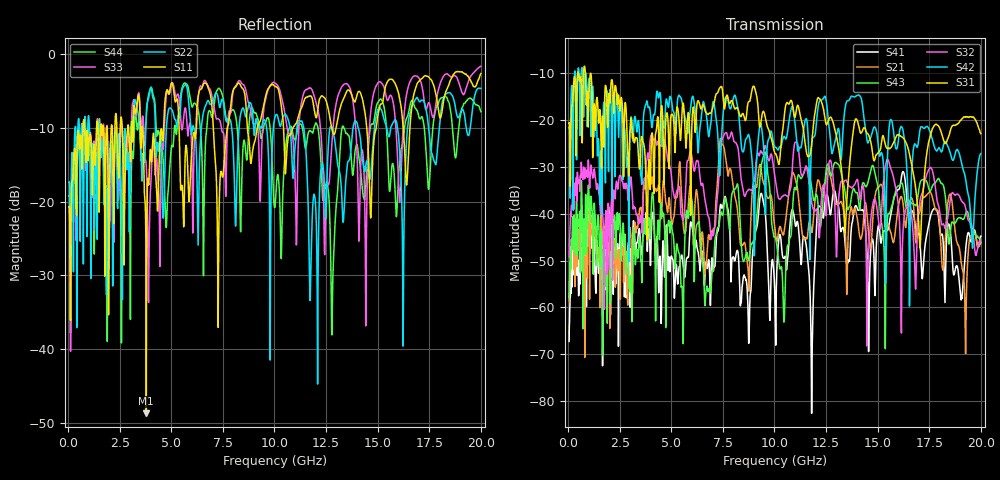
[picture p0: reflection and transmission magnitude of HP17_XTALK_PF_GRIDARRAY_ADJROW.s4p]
# MHz S MA R 50.00
! FREQ  S11  S12  S13  S14
!  S21  S22  S23  S24
!  S31  S32  S33  S34
!  S41  S42  S43  S44
!  MAG  ANG  MAG  ANG  MAG  ANG  MAG  ANG
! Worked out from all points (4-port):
!   1996 points, 50 MHz to 20 GHz, reference 50 ohm
!   strongest paths, dB at 50 MHz, 5.04 GHz, 10.03 GHz, 15.02 GHz, 20 GHz:
!     S31: -20.7, -18.7, -27.1, -27.0, -22.9
!     S42: -21.5, -16.9, -25.7, -25.0, -27.1
!     S32: -49.2, -33.5, -32.4, -40.8, -45.7
!     S43: -58.0, -43.3, -45.0, -34.3, -46.2
!     S21: -58.6, -42.3, -43.4, -34.4, -46.0
!     S41: -67.3, -49.4, -59.9, -42.8, -44.8
!   lowest |S11| = -48.7 dB at 3.79 GHz (marker M1), VSWR 1.01, Z = 50.3 - j0.255 ohm
!   |S11| at or under -10 dB: 3.612 GHz to 4.63 GHz (1.018 GHz wide, 24.7 % of centre); 5.379 GHz to 6.2 GHz (821.5 MHz wide, 14.2 % of centre); 7.037 GHz to 7.717 GHz (680.1 MHz wide, 9.22 % of centre)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
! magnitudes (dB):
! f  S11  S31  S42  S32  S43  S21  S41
! 50 MHz  -20.7  -20.7  -21.5  -49.2  -58.0  -58.6  -67.3
! 3.79 GHz  -48.7  -36.7  -16.3  -28.8  -41.0  -30.7  -39.7
! 10.88 GHz  -10.1  -16.9  -17.1  -29.0  -38.6  -31.1  -39.2
! 11.81 GHz  -5.8  -24.7  -24.8  -37.8  -34.6  -44.0  -77.7
! 12.8 GHz  -10.4  -20.0  -27.1  -30.6  -31.0  -34.0  -37.0
! 17.04 GHz  -3.5  -46.9  -22.3  -37.5  -33.6  -39.6  -45.5
! 20 GHz  -2.6  -22.9  -27.1  -45.7  -46.2  -46.0  -44.8
